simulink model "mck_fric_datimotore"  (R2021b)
settings: Solver=VariableStepAuto  StartTime=0.0  StopTime=20  RelTol=1e-3
undefined symbols (not defined in the file or in its folder): BLDC, dynamics
libraries: fl_lib x9, nesl_utility x4

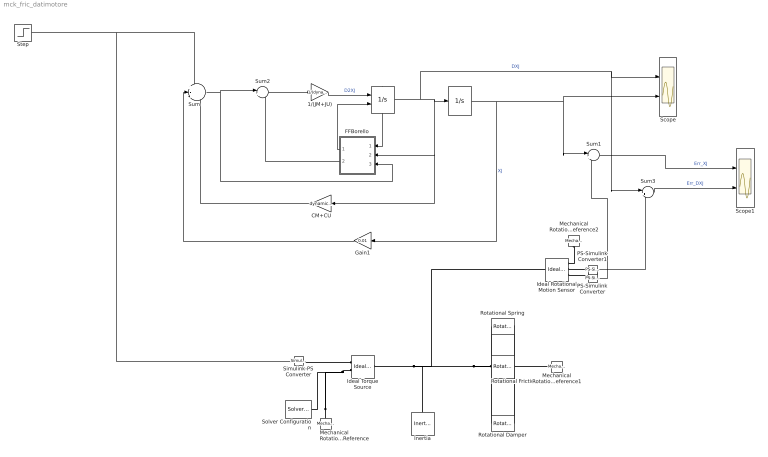
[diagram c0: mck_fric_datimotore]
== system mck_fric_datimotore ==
  " " : Integrator  ExternalReset=rising  ShowStatePort=on
  "  " : Integrator  UpperSaturationLimit=dynamics.ThUmax/dynamics.tau  LowerSaturationLimit=dynamics.ThUmin/dynamics.tau
  1/(JM+JU) : Gain  Gain=1/(dynamics.JM+dynamics.JU)
  CM+CU : Gain  Gain=dynamics.CM+dynamics.CU
  FFBorello : Subsystem
  Gain1 : Gain  Gain=0.01
  Ideal Rotational Motion Sensor : fl_lib/Mechanical/Mechanical Sensors/Ideal Rotational Motion Sensor  wrap_angle=simscape.enum.onoff.off  offset=0 rad
  Ideal Torque Source : fl_lib/Mechanical/Mechanical Sources/Ideal Torque Source
  Inertia : fl_lib/Mechanical/Rotational Elements/Inertia  inertia=dynamics.JM+dynamics.JU kg*m^2  num_ports=foundation.enum.numPorts2.one  w_specify=off  w_priority=High  w=0 rad/s  w_nominal_specify=off  w_nominal_unit=rad/s  w_nominal_value=1  t_specify=off  t_priority=None  t=0 N*m  t_nominal_specify=off  t_nominal_unit=N*m  t_nominal_value=1
  Mechanical Rotational Reference : fl_lib/Mechanical/Rotational Elements/Mechanical Rotational Reference
  Mechanical Rotational Reference1 : fl_lib/Mechanical/Rotational Elements/Mechanical Rotational Reference
  Mechanical Rotational Reference2 : fl_lib/Mechanical/Rotational Elements/Mechanical Rotational Reference
  PS-Simulink Converter : nesl_utility/PS-Simulink Converter  PhysicalDomain=network_engine_domain  SubClassName=ps_output  LeftPortType=input  RightPortType=output  PseudoPeriodic=off  Frequencies=[]  Unit=inherit  AffineConversion=off
  PS-Simulink Converter1 : nesl_utility/PS-Simulink Converter  PhysicalDomain=network_engine_domain  SubClassName=ps_output  LeftPortType=input  RightPortType=output  PseudoPeriodic=off  Frequencies=[]  Unit=inherit  AffineConversion=off
  Rotational Damper : fl_lib/Mechanical/Rotational Elements/Rotational Damper  D=dynamics.CM+dynamics.CU N*m/(rad/s)  w_specify=off  w_priority=None  w=0 rad/s  w_nominal_specify=off  w_nominal_unit=rad/s  w_nominal_value=1  t_specify=off  t_priority=None  t=0 N*m  t_nominal_specify=off  t_nominal_unit=N*m  t_nominal_value=1
  Rotational Friction : fl_lib/Mechanical/Rotational Elements/Rotational Friction  brkwy_trq=(dynamics.friction.FSTm+dynamics.friction.FSTu)*BLDC.TMM N*m  brkwy_vel=0.00001201 rad/s  Col_trq=(dynamics.friction.FDTm+dynamics.friction.FDTu)*BLDC.TMM N*m  visc_coef=0 N*m/(rad/s)  w_specify=off  w_priority=None  w=0 rad/s  w_nominal_specify=off  w_nominal_unit=rad/s  w_nominal_value=1  t_specify=off  t_priority=None  t=0 N*m  t_nominal_specify=off  t_nominal_unit=N*m  t_nominal_value=1
  Rotational Spring : fl_lib/Mechanical/Rotational Elements/Rotational Spring  spr_rate=0.01 N*m/rad  w_specify=off  w_priority=None  w=0 rad/s  w_nominal_specify=off  w_nominal_unit=rad/s  w_nominal_value=1  t_specify=off  t_priority=None  t=0 N*m  t_nominal_specify=off  t_nominal_unit=N*m  t_nominal_value=1  phi_specify=off  phi_priority=High  phi=0 rad  phi_nominal_specify=off  phi_nominal_unit=rad  phi_nominal_value=1
  Scope : Scope  NumInputPorts=2
  Scope1 : Scope  NumInputPorts=2
  Simulink-PS Converter : nesl_utility/Simulink-PS Converter  PhysicalDomain=network_engine_domain  SubClassName=ps_input  LeftPortType=input  RightPortType=output  PseudoPeriodic=off  Frequencies=[]  NoiseDistribution=none  NoiseParameters=[]  Unit=1  AffineConversion=off  FilteringAndDerivatives=provide  SimscapeFilterOrder=1  InputFilterTimeConstant=0.001  UdotUserProvided=0
  Solver Configuration : nesl_utility/Solver Configuration  PhysicalDomain=network_engine_domain  SubClassName=solver  LeftPortType=input  RightPortType=generic  Tones=[]  Harmonics=[]  SimulateNoise=off  Profile=off  UseLocalSampling=off  EnableSwitchedLinearOptims=on  FrequencyDomain=off  UseCCode=off  RelTol=0.001  AbsTol=1e-06  MinStep=1e-09  ToWorkspace=off  RevertToSquareIcSolve=off  NumHomotopyIterations=100  PhasorMode=off  PhasorModeNumHarmonics=1  DoDC=off  ResidualTolerance=1e-09  UseLocalSolver=off  LocalSolverChoice=NE_BACKWARD_EULER_ADVANCER  LocalSolverSampleTime=0.001  DoFixedCost=off  MaxNonlinIter=3  MaxModeIter=2  ComputeImpulses=off  ImpulseIterations=2  LinearAlgebra=auto  EquationFormulation=NE_TIME_EF  DelaysMemoryBudget=1024  AutomaticFiltering=on  FilteringTimeConstant=0.001  PartitionStorageMethod=AS_NEEDED  PartitionMemoryBudget=1024  PartitionMethod=ROBUST
  Step : Step  Time=10  Before=0.17  After=-0.17  SampleTime=0
  Sum : Sum  Inputs=+--
  Sum1 : Sum  Inputs=|+-
  Sum2 : Sum  Inputs=|+-
  Sum3 : Sum  Inputs=|+-
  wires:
  FFBorello/2(TF) -> Sum2/2
  " "/1 -> Sum3/1, Scope/1, "  "/1, CM+CU/1, FFBorello/2(DXJ)  "DXJ"
  " "/State -> FFBorello/1(DXJ SP)
  FFBorello/1(Reset_DXJ) -> " "/2
  Gain1/1 -> Sum/2
  Sum1/1 -> Scope1/1  "Err_XJ"
  Sum3/1 -> Scope1/2  "Err_DXJ"
  CM+CU/1 -> Sum/3
  PS-Simulink Converter1/1 -> Sum3/2
  1/(JM+JU)/1 -> " "/1  "D2XJ"
  Sum2/1 -> 1/(JM+JU)/1
  Step/1 -> Simulink-PS Converter/1, Sum/1
  "  "/1 -> Sum1/1, Scope/2, Gain1/1  "XJ"
  Sum/1 -> FFBorello/3(Act Torque), Sum2/1
  PS-Simulink Converter/1 -> Sum1/2
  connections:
  Ideal Torque Source/LConn1 -- Ideal Rotational Motion Sensor/LConn1 -- Inertia/LConn1 -- Rotational Damper/LConn1 -- Rotational Spring/LConn1 -- Rotational Friction/LConn1
  Ideal Torque Source/RConn2 -- Mechanical Rotational Reference/LConn1 -- Solver Configuration/RConn1
  Rotational Spring/RConn1 -- Mechanical Rotational Reference1/LConn1 -- Rotational Damper/RConn1 -- Rotational Friction/RConn1
  Simulink-PS Converter/RConn1 -- Ideal Torque Source/RConn1
  PS-Simulink Converter/LConn1 -- Ideal Rotational Motion Sensor/RConn3
  Mechanical Rotational Reference2/LConn1 -- Ideal Rotational Motion Sensor/RConn1
  PS-Simulink Converter1/LConn1 -- Ideal Rotational Motion Sensor/RConn2

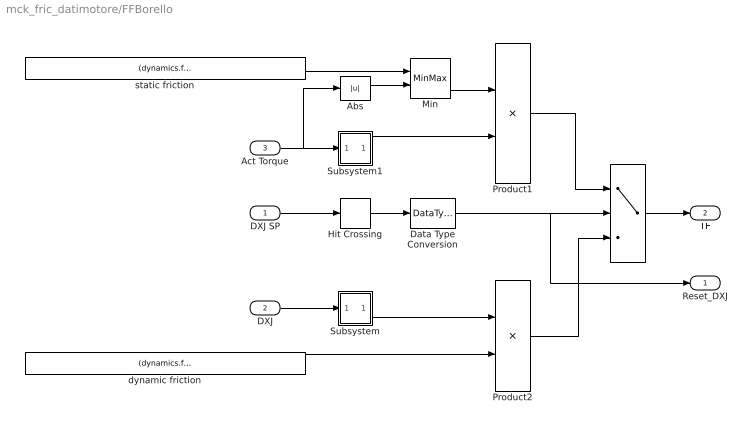
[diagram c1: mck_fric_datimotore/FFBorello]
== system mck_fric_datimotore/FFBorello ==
  DXJ SP : Inport
  DXJ : Inport  Port=2
  Act Torque : Inport  Port=3
  "   " : Switch  Threshold=0.5
  Abs : Abs
  Data Type Conversion : DataTypeConversion  OutDataTypeStr=double
  Hit Crossing : HitCross
  Min : MinMax  Inputs=2  InputSameDT=on  SaturateOnIntegerOverflow=on
  Product1 : Product  InputSameDT=on  RndMeth=Zero  SaturateOnIntegerOverflow=on
  Product2 : Product  InputSameDT=on  RndMeth=Zero  SaturateOnIntegerOverflow=on
  Subsystem : Subsystem
  Subsystem1 : Subsystem
  dynamic friction : Constant  Value=(dynamics.friction.FDTm+dynamics.friction.FDTu)*BLDC.TMM
  static friction : Constant  Value=(dynamics.friction.FSTm+dynamics.friction.FSTu)*BLDC.TMM
  Reset_DXJ : Outport
  TF : Outport  Port=2
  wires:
  Product2/1 -> "   "/3
  DXJ/1 -> Subsystem/1(In1)
  "   "/1 -> TF/1
  Product1/1 -> "   "/1
  Min/1 -> Product1/1
  Act Torque/1 -> Subsystem1/1(In1), Abs/1
  Abs/1 -> Min/2
  Hit Crossing/1 -> Data Type Conversion/1
  Subsystem/1(Out1) -> Product2/1
  Subsystem1/1(Out1) -> Product1/2
  Data Type Conversion/1 -> "   "/2, Reset_DXJ/1
  DXJ SP/1 -> Hit Crossing/1
  static friction/1 -> Min/1
  dynamic friction/1 -> Product2/2

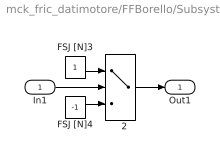
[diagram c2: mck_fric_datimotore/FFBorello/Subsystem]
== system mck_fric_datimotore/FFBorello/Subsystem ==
  In1 : Inport
  "   2" : Switch
  FSJ [N]3 : Constant
  FSJ [N]4 : Constant  Value=-1
  Out1 : Outport
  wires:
  FSJ [N]3/1 -> "   2"/1
  FSJ [N]4/1 -> "   2"/3
  In1/1 -> "   2"/2
  "   2"/1 -> Out1/1

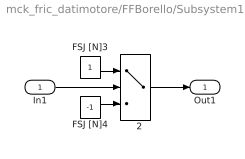
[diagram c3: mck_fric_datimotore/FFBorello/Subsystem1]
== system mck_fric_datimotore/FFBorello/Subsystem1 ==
  In1 : Inport
  "   2" : Switch
  FSJ [N]3 : Constant
  FSJ [N]4 : Constant  Value=-1
  Out1 : Outport
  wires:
  FSJ [N]3/1 -> "   2"/1
  FSJ [N]4/1 -> "   2"/3
  In1/1 -> "   2"/2
  "   2"/1 -> Out1/1
